(* Logix 5000 AddOnInstructionDefinition export AOI_ISC_OutDataConversion; software revision 32.02 *)

ADD_ON_INSTRUCTION AOI_ISC_OutDataConversion   (* revision 1.0 *)
// Output data conversions for ISC CAM IDL V2.0
VAR_OUTPUT
   OutputWord1 : INT; {required}   // Output Word 1 Data Mapping for Communication
        .8   // Run Mode Internal ISC CAM
        .9   // Run Mode External PLC
   OutputWord3 : INT; {access Read Only, required}   // Output Word 3 Data Mapping for Communication
   OutputWord4 : INT; {access Read Only, required}   // Output Word 4 Data Mapping for Communication
   OutputWord5 : INT; {access Read Only, required}   // Output Word 5 Data Mapping for Communication
   OutputWord6 : INT; {required}   // Output Word 6 Data Mapping for Communication
   OutputWord7 : INT; {required}   // Output Word 7 Data Mapping for Communication
        .2   // Active Carryway 1 Enable Left
        .3   // Active Carryway 1 Enable Right
        .4   // Active Carryway 2 Enable Left
        .5   // Active Carryway 2 Enable Right
        .6   // Active Carryway 3 Enable Left
        .7   // Active Carryway 3 Enable Right
   OutputWord12 : INT; {access Read Only, required}   // Output Word 12 Data Mapping for Communication
        .8   // Parameter Read Value Trigger
        .9   // Parameter Write Value Trigger
END_VAR
VAR_INPUT
   ProductDest : INT; {required}   // Product Destination
   RunModeInternal : BOOL; {required}   // Run Mode Internal ISC CAM Logic Control
   RunModeExternal : BOOL; {required}   // Run Mode External PLC Logic Control
   ProductsDest0 : INT; {required}   // Number of Products to Destination 0
   ProductsDest1 : INT; {required}   // Number of Products to Destination 1
   ProductsDest2 : INT; {required}   // Number of Products to Destination 2
   ProductsDest3 : INT; {required}   // Number of Products to Destination 3
   ProductsDest4 : INT; {required}   // Number of Products to Destination 4
   ProductsDest5 : INT; {required}   // Number of Products to Destination 5
   ProductsDest6 : INT; {required}   // Number of Products to Destination 6
   EnableLeftCarryway1 : BOOL; {required}   // Active Carryway 1 Enable Left
   EnableRightCarryway1 : BOOL; {required}   // Active Carryway 1 Enable Right
   EnableLeftCarryway2 : BOOL; {required}   // Active Carryway 2 Enable Left
   EnableRightCarryway2 : BOOL; {required}   // Active Carryway 2 Enable Right
   EnableLeftCarryway3 : BOOL; {required}   // Active Carryway 3 Enable Left
   EnableRightCarryway3 : BOOL; {required}   // Active Carryway 3 Enable Right
   OverrideCarrywayPointer : INT; {required}   // Override Active Carryway Pointer
   ParameterGroup : INT; {required}   // Parameter Group
   ParameterRead : BOOL; {required}   // Parameter Read Trigger
   ParameterWrite : BOOL; {required}   // Parameter Write Trigger
END_VAR
VAR
   BTDT_OW1B0 : FBD_BIT_FIELD_DISTRIBUTE := (Length := 1); {access None}
   BTDT_OW3B0 : FBD_BIT_FIELD_DISTRIBUTE := (Length := 1); {access None}
   BTDT_OW4B0 : FBD_BIT_FIELD_DISTRIBUTE := (Length := 1); {access None}
   BTDT_OW5B0 : FBD_BIT_FIELD_DISTRIBUTE := (Length := 1); {access None}
   BTDT_OW6B0 : FBD_BIT_FIELD_DISTRIBUTE := (Length := 1); {access None}
   BTDT_OW7B1 : FBD_BIT_FIELD_DISTRIBUTE := (Length := 1); {access None}
   BTDT_OW12B0 : FBD_BIT_FIELD_DISTRIBUTE := (Length := 1); {access None}
   BTDT_OW3B1 : FBD_BIT_FIELD_DISTRIBUTE := (Length := 1); {access None}
   BTDT_OW4B1 : FBD_BIT_FIELD_DISTRIBUTE := (Length := 1); {access None}
   BTDT_OW5B1 : FBD_BIT_FIELD_DISTRIBUTE := (Length := 1); {access None}
END_VAR

ROUTINE Logic   (* structured text *)
   //Output Word 1 Mapping
   BTDT_OW1B0.Source:=ProductDest;
   BTDT_OW1B0.SourceBit:=0;
   BTDT_OW1B0.DestBit:=0;
   BTDT_OW1B0.Length:=8;
   BTDT_OW1B0.Target:=OutputWord1;
   BTDT(BTDT_OW1B0);
   OutputWord1:=BTDT_OW1B0.Dest;
   
   OutputWord1.8:=RunModeInternal;
   OutputWord1.9:=RunModeExternal;
   
   //Output Word 3 Mapping
   BTDT_OW3B0.Source:=ProductsDest0;
   BTDT_OW3B0.SourceBit:=0;
   BTDT_OW3B0.DestBit:=0;
   BTDT_OW3B0.Length:=8;
   BTDT_OW3B0.Target:=OutputWord3;
   BTDT(BTDT_OW3B0);
   OutputWord3:=BTDT_OW3B0.Dest;
   
   BTDT_OW3B1.Source:=ProductsDest1;
   BTDT_OW3B1.SourceBit:=0;
   BTDT_OW3B1.DestBit:=8;
   BTDT_OW3B1.Length:=8;
   BTDT_OW3B1.Target:=OutputWord3;
   BTDT(BTDT_OW3B1);
   OutputWord3:=BTDT_OW3B1.Dest;
   
   //Output Word 4 Mapping
   BTDT_OW4B0.Source:=ProductsDest2;
   BTDT_OW4B0.SourceBit:=0;
   BTDT_OW4B0.DestBit:=0;
   BTDT_OW4B0.Length:=8;
   BTDT_OW4B0.Target:=OutputWord4;
   BTDT(BTDT_OW4B0);
   OutputWord4:=BTDT_OW4B0.Dest;
   
   BTDT_OW4B1.Source:=ProductsDest3;
   BTDT_OW4B1.SourceBit:=0;
   BTDT_OW4B1.DestBit:=8;
   BTDT_OW4B1.Length:=8;
   BTDT_OW4B1.Target:=OutputWord4;
   BTDT(BTDT_OW4B1);
   OutputWord4:=BTDT_OW4B1.Dest;
   
   //Output Word 5 Mapping
   BTDT_OW5B0.Source:=ProductsDest4;
   BTDT_OW5B0.SourceBit:=0;
   BTDT_OW5B0.DestBit:=0;
   BTDT_OW5B0.Length:=8;
   BTDT_OW5B0.Target:=OutputWord5;
   BTDT(BTDT_OW5B0);
   OutputWord5:=BTDT_OW5B0.Dest;
   
   BTDT_OW5B1.Source:=ProductsDest5;
   BTDT_OW5B1.SourceBit:=0;
   BTDT_OW5B1.DestBit:=8;
   BTDT_OW5B1.Length:=8;
   BTDT_OW5B1.Target:=OutputWord5;
   BTDT(BTDT_OW5B1);
   OutputWord5:=BTDT_OW5B1.Dest;
   
   //Output Word 6 Mapping
   BTDT_OW6B0.Source:=ProductsDest6;
   BTDT_OW6B0.SourceBit:=0;
   BTDT_OW6B0.DestBit:=0;
   BTDT_OW6B0.Length:=8;
   BTDT_OW6B0.Target:=OutputWord6;
   BTDT(BTDT_OW6B0);
   OutputWord6:=BTDT_OW6B0.Dest;
   
   //Output Word 7 Mapping
   OutputWord7.2:=EnableLeftCarryway1;
   OutputWord7.3:=EnableRightCarryway1;
   OutputWord7.4:=EnableLeftCarryway2;
   OutputWord7.5:=EnableRightCarryway2;
   OutputWord7.6:=EnableLeftCarryway3;
   OutputWord7.7:=EnableRightCarryway3;
   
   BTDT_OW7B1.Source:=OverrideCarrywayPointer;
   BTDT_OW7B1.SourceBit:=0;
   BTDT_OW7B1.DestBit:=8;
   BTDT_OW7B1.Length:=8;
   BTDT_OW7B1.Target:=OutputWord7;
   BTDT(BTDT_OW7B1);
   OutputWord7:=BTDT_OW7B1.Dest;
   
   //Output Word 12 Mapping
   BTDT_OW12B0.Source:=ParameterGroup;
   BTDT_OW12B0.SourceBit:=0;
   BTDT_OW12B0.DestBit:=0;
   BTDT_OW12B0.Length:=8;
   BTDT_OW12B0.Target:=OutputWord12;
   BTDT(BTDT_OW12B0);
   OutputWord12:=BTDT_OW12B0.Dest;
   
   OutputWord12.8:=ParameterRead;
   OutputWord12.9:=ParameterWrite;
END_ROUTINE
END_ADD_ON_INSTRUCTION
